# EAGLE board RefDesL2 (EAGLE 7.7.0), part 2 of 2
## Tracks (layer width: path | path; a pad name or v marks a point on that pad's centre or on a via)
AGND
  Top 0.152: 29.87,30.63 U2.A6 29.26,31.19 29.26,32 29.62,32.37 30.81,32.37 | C13.2 C15.2 C14.2 26.75,33.25 26.98,33.02 28.35,33.02 28.5,33.17 28.5,33.98 28.93,34.42 U2.A9 30.35,34.42 30.48,34.29 30.48,34.28 30.54,34.22 30.54,32.63 | 30.81,32.37 34.14,32.37 U2.E8 | 30.54,32.63 30.81,32.37 | 30.54,32.63 30.54,32.37
ANLG0  (via drill 0.3 pad 0.61)
  Top 0.152: v26.06,46.63 25.6,46.63 24.69,47.55 24.69,54.56 24.13,55.12 X6.1 | U2.B6 30.5,31.22 v30.5,31.47
  Bottom 0.152: v26.06,46.63 25.6,46.18 25.6,32.61 26.98,31.24 30.28,31.24 v30.5,31.47
CGND
  Top 0.381: X3.CGND1 X3.CGND2 X3.CGND3 X3.CGND4 | 17.42,15.27 X5.CGND5 | X5.CGND5 17.43,14.39 18.54,13.28 21.39,13.28 22.1,12.57 22.1,11.11 X5.CGND4 | 0.99,12.39 0.99,12.4 X5.CGND1 9.37,12.4 9.86,12.88 9.86,14.86 10.26,15.27 11.42,15.27 X5.CGND6 X5.CGND5
  Top 0.762: R2.1 4.7,63.88
  pour Top: 0,44.45 0,69.85 63.5,69.85 63.5,38.1 62.23,38.1 62.23,41.53 57.91,41.53 57.91,43.81 62.23,43.81 62.23,49.99 57.91,49.99 57.91,52.32 62.23,52.32 62.23,63.5 58.45,63.5 57.15,64.72 57.15,68.58 6.35,68.58 6.35,64.77 5.08,63.5 1.27,63.5 1.27,44.45
  pour Top: 0,44.45 1.27,44.45 1.27,6.35 5.08,6.35 6.35,5.08 6.35,2.03 23.44,2.03 23.44,1.27 41.53,1.27 41.53,11.66 42.27,12.4 44.42,12.4 45.77,11.13 54.56,11.13 55.75,12.4 57.71,12.4 58.47,11.43 62.23,11.43 62.23,38.1 63.5,38.1 63.5,0 0,0
  pour Bottom: 0,44.45 0,69.85 63.5,69.85 63.5,38.1 62.23,38.1 62.23,63.5 58.42,63.5 57.15,64.77 57.15,68.58 6.35,68.58 6.35,64.77 5.08,63.5 1.27,63.5 1.27,44.45
  pour Bottom: 0,44.45 1.27,44.45 1.27,6.35 5.08,6.35 6.35,5.08 6.35,1.27 41.53,1.27 41.53,11.66 42.29,12.4 44.42,12.4 45.75,11.15 45.77,11.13 54.56,11.13 54.56,11.1 55.75,12.4 57.68,12.4 58.45,11.43 62.23,11.43 62.23,38.1 63.5,38.1 63.5,0 0,0
ECAP_PWM0  (via drill 0.3 pad 0.61)
  Top 0.152: v29.34,37.52 29.01,37.85 25.2,37.85 24.84,37.49 24.84,32.97 24.13,32.26 X6.16 | U2.C18 31.8,45.26 v31.7,45.26
  Bottom 0.152: v31.7,45.26 31.7,40.39 33.68,38.41 33.68,37.03 32.31,35.66 30.63,35.66 29.34,36.96 v29.34,37.52
EMMC_RSTN  (via drill 0.3)
  Top 0.152: U2.R14 47.62,40.26 46.99,39.62 46.99,37.85 46.74,37.59 45.97,37.59 45.72,37.34 v45.72,32.64 | U9.K5 v27.97,9.34 | v27.96,9.35 v27.97,9.34 | R45.1 27.91,9.4 v27.97,9.34
  Bottom 0.152: v27.97,9.34 28.78,10.15 28.78,16.97 29.39,17.58 36.85,17.58 39.17,19.89 39.17,24.31 40.51,25.65 42.67,25.65 45.34,28.32 45.34,31.75 45.72,32.13 v45.72,32.64
GND  (via drill 0.3, 0.3 pad 0.61, 0.38, 0.38 pad 0.61, 0.76)
  Top 0.152: v44.04,57.76 43.89,57.76 43.23,58.42 C8.2 | v27.05,58.29 26.8,58.04 R26.1 | v29.26,45.41 29.26,45.72 29.39,45.85 U2.A18 | v26.92,25.02 27,25.09 R6.2 | U2.A1 29.26,24.84 v29.11,24.84 | U9.G5 30.71,10.84 | U9.N5 U9.P6 31.27,7.28 v31.27,6.55 | v30.48,6.55 30.48,7.07 U9.P4 | v23.24,16.64 C19.2 | U9.N2 28.33,7.84 27.94,8.23 v27.94,8.26 | U1.1 57.94,16.1 57.58,15.75 R1.1 v57.58,14.53 | v56.01,17.02 U1.TH | U9.C4 30.2,11.03 | R62.1 v57.25,50.42 | R61.1 v55.5,50.42 | v30.38,65.58 31.04,65.58 R39.1 | v45.59,45.21 45.72,45.21 U2.P17
  Top 0.254: U3.4 50.92,16.54 50.98,16.54 | C2.2 51,16.61 | v55.12,47.73 55.55,47.3 U5.4 | U9.H10 32.97,10.34 32.72,10.59 v31.95,10.59 | v31.95,10.59 31.14,10.59 30.89,10.84 U9.G5 30.38,10.84 30.2,11.02 30.2,11.03 | U9.K8 32.2,9.51 31.96,9.76 v31.96,10.59 v31.95,10.59 | U9.E7 31.7,11.76 31.95,11.51 v31.95,10.59 | 50.98,16.61 C2.2 | v51.92,16.54 50.98,16.54 | 50.98,16.54 C2.2 | R15.2 R57.2 | R57.2 R58.2 R59.1 R60.1 v53.59,50.42 | v48.26,50.42 R57.2
  Top 0.305: v13.46,67.44 12.21,67.44 RESET.4 | POWER.1 12.27,62.33 v13.56,62.33 | 16.92,60.72 BTN2.4 17,60.73 v15.85,60.73 | 16.93,65.8 BTN1.4 17,65.81 v15.85,65.81 | R7.1 v42.06,20.17 | R16.1 v44.04,20.17 | R23.1 v46.02,20.17 | R18.1 v48.01,20.17 | R10.1 v55.93,20.17 | U4.3 25.11,66.67 v24.26,66.67 | U6.1 24.38,60.33 v23.09,60.33 | X4.8 v36.58,64.77 | X4.4 v34.04,64.77 | X4.16 v41.66,64.77 | X4.20 v44.2,64.77 | C10.2 38.35,58.5 v38.35,59.44 | v51.97,20.17 R14.1 | C18.1 v20.95,19.81
  Top 0.381: U2.W3 U2.W2 v52.07,24.89 U2.V1 | RESET.2 RESET.4 | POWER.3 POWER.1 | BTN2.4 BTN2.2 | BTN1.4 BTN1.2 | X4.8 X4.10 X4.12 | R11.1 R14.1 R13.1 R12.1 | R7.1 R21.1 | R22.1 R23.1 R17.1 | R9.1 R10.1 | X3.GND | v30.35,2.92 C16.1 | v20.19,14.73 18.65,14.73 X5.GND | C9.1 v4.06,16.64 | C17.1 22.17,15.9 v21.46,15.9 | C11.2 v5.33,11.56 | C21.1 38.41,3.3 v37.72,3.3 | U7.2 v5.08,18.67 | v21.21,3.3 21.27,3.36 X5.6 | C20.1 40.72,6.27 v40.77,6.22 | C3.2 55.35,41.17 v55.12,41.4 | C12.2 v16,18.41
  Top 0.762: R2.2 v2.92,60.2
  other vias: 57.78,48.56 39.37,47.75 38.13,37.59 40.64,37.59 43.18,37.59 43.18,40.13 43.18,35 41.91,35.05 40.64,35.05 39.37,35.05 38.13,35.05 39.37,32.51 40.64,32.51 41.91,32.51 43.18,32.51 41.91,38.73 40.64,47.75 41.91,47.75 35.69,47.75 53.34,47.75 53.34,38.86 53.34,36.32 38.13,36.32 38.13,33.76 40.64,33.78 40.64,36.32 53.39,43.97 53.39,45.21 48.26,47.75 53.14,32.46 39.4,31.24 40.64,31.24 43.18,31.24 44.45,36.32 44.45,40.13 59.97,12.95 61.06,12.95 55.24,17.78 56.01,17.78 55.24,17.02 53.14,33.81 57.78,49.28
  pour Route15: -2.54,72.39 66.04,72.39 66.04,-2.54 -2.54,-2.54
  pour Top: 45.09,41.4 43.18,41.4 43.18,40.13 41.91,40.13 41.91,38.86 37.34,38.86 37.34,37.59 36.83,37.59 36.83,33.78 36.2,33.78 36.2,32.51 38.1,32.51 38.1,29.97 44.45,29.97 44.45,31.24 45.09,31.24 45.09,37.59 44.45,37.59 44.45,40.13 45.09,40.13
  pour Top (rank 2): 52.7,29.34 53.34,29.34 53.34,31.75 54.36,31.75 54.36,32 53.34,32 53.34,35.69 53.98,35.69 53.98,48.39 52.7,48.39 52.7,47.75 48.9,47.75 48.9,48.39 34.92,48.39 34.92,47.12 50.29,47.12 51.44,45.85 52.7,45.85
  pour Top (no thermals): 59.05,15.62 61.85,15.62 61.85,12.57 59.05,12.57
  pour Top (no thermals): 57.15,49.61 58.42,49.61 58.42,48.64 58.55,48.51 60.07,48.51 60.07,48.01 58.46,48.01 58.17,48.29 57.16,48.29
I2C0_SCL  (via drill 0.3 pad 0.61)
  Top 0.152: U2.C20 v31.7,49.07 32.18,49.55 R4.1 | v33.07,43.89 32.97,43.89 U2.C16 31.9,42.82 31.9,41.53 31.62,41.25 30.78,41.25 30.48,40.95 30.48,40.51 30.25,40.28 29.36,40.28 28.83,39.75 4.12,39.75 1.93,37.57 1.93,20.42 2.67,19.68 3.84,19.68 3.85,19.67 U7.1
  Bottom 0.152: v33.07,43.89 32.77,44.2 32.77,46.33 31.7,47.4 v31.7,49.07
I2C0_SDA
  Top 0.152: U2.C19 33.07,46.43 33.07,46.33 | 33.07,46.33 33.07,46.18 | 33.07,46.18 33.07,46.02 | 33.07,46.02 33.07,45.26 U2.C17 31.6,43.79 31.6,41.73 31.42,41.55 29.94,41.55 28.52,40.13 4.06,40.13 1.63,37.69 1.63,18.19 2.03,17.78 3.84,17.78 3.85,17.77 U7.3 | 33.38,46.33 33.53,46.48 33.83,46.48 34.29,46.94 34.29,47.55 34.14,47.7 33.5,47.7 33.17,48.03 33.17,49.91 33.35,50.09 R3.1 | 33.38,46.33 33.22,46.18 | 33.22,46.18 33.07,46.02 | 33.07,46.18 33.22,46.18 | 33.07,46.33 33.38,46.33
I2C1_SCL  (via drill 0.3)
  Top 0.152: v35.53,45.14 34.98,44.58 U2.E17 | X6.12 10.72,30.15 5.51,30.15 5.08,29.72 I2C1_SCL.TP
  Bottom 0.152: v35.53,45.14 35.53,45.62 36.17,46.25 36.17,47.02 36.35,47.19 36.35,48.18 35.41,49.12 35.41,55.55 35.74,55.88 37.36,55.88 38.02,56.54 44.65,56.54 45.31,57.2 45.31,62.33 45.03,62.61 45.03,65.28 43.84,66.47 30.02,66.47 21.61,58.06 11.05,58.06 8.99,56.01 8.99,31.52 9.6,30.91 11.48,30.91 X6.12
I2C1_SDA  (via drill 0.3)
  Top 0.152: U2.E18 v35.56,46.48 | X6.11 8.53,30.5 3.58,30.5 3.05,29.97 I2C0_SDA.TP
  Bottom 0.152: v35.56,46.48 35.1,46.94 35.1,55.7 35.61,56.21 37.19,56.21 37.82,56.84 44.48,56.84 44.98,57.35 44.98,62.13 44.73,62.38 44.73,65.13 43.69,66.17 30.2,66.17 21.74,57.71 12.42,57.71 11.66,56.95 11.66,33.63 X6.11
JTAG_EMU0  (via drill 0.3 pad 0.61)
  Top 0.152: 40.54,61.58 X4.13 40.39,59.56 40.56,59.38 R27.1 40.56,58.09 v40.23,57.76 | U2.C14 32.61,41 33.2,41 33.66,41.45 33.86,41.45 34.14,41.73 34.14,45.06 v34.27,45.19
  Bottom 0.152: v40.23,57.76 37.64,57.76 36.73,56.84 35.2,56.84 34.49,56.13 34.49,45.41 v34.27,45.19
JTAG_EMU1  (via drill 0.3 pad 0.61)
  Top 0.152: v33.05,41.6 32.77,41.6 32.61,41.45 32.31,41.45 31.62,40.77 U2.B14 | X4.14 v40.39,64.92 41.15,64.16 44.5,64.16 45.16,64.82 R42.1
  Bottom 0.152: v33.05,41.6 33.22,41.6 33.98,42.37 33.98,44.35 33.38,44.96 33.38,46.63 33.07,46.94 33.07,55.63 34.59,57.15 36.42,57.15 37.8,58.52 43.99,58.52 44.37,58.9 44.37,61.77 43.81,62.33 41,62.33 40.39,62.94 v40.39,64.92
JTAG_EMU2  (via drill 0.3 pad 0.61)
  Top 0.152: v23.32,41.91 23.32,41.76 23.98,41.1 25.73,41.1 R44.2 | v42.93,59.44 X4.17
  Bottom 0.152: v23.32,41.91 23.32,48.77 25.3,50.75 25.3,59.33 26.16,60.2 36.42,60.2 36.73,60.5 41.86,60.5 v42.93,59.44
JTAG_EMU3  (via drill 0.3 pad 0.61)
  Top 0.152: v42.93,64.9 X4.18 | U2.D14 33.93,41.05 v34.27,41.05
  Bottom 0.152: v34.27,41.05 34.27,41.66 34.44,41.83 34.44,44.12 34.8,44.48 34.8,55.88 35.46,56.54 37.03,56.54 37.64,57.15 44.35,57.15 44.68,57.48 44.68,62 42.93,63.75 v42.93,64.9
JTAG_TCK  (via drill 0.3 pad 0.61)
  Top 0.152: 29.87,38.25 U2.A12 29.18,38.23 v28.96,38.46 | v37.11,59.44 37.49,59.44 37.85,59.79 X4.9
  Top 0.381: X4.9 X4.11
  Bottom 0.152: v37.11,59.44 36.73,59.44 36.27,59.89 31.55,59.89 28.19,56.54 28.19,46.63 26.21,44.65 26.21,40.69 26.82,40.08 28.19,40.08 28.96,39.32 v28.96,38.46
JTAG_TDI  (via drill 0.3 pad 0.61)
  Top 0.152: v35.36,58.52 34.04,59.84 X4.3 | U2.B11 31.7,37.54 v31.7,37.64
  Bottom 0.152: v31.7,37.64 31.7,38.86 30.79,39.78 29.41,39.78 28.5,40.69 27.13,40.69 26.82,41 26.82,44.35 28.8,46.33 28.8,56.24 31.39,58.83 34.59,58.83 34.9,58.52 v35.36,58.52
JTAG_TDO  (via drill 0.3 pad 0.61)
  Top 0.152: v36.12,59.28 36.58,59.74 X4.7 | U2.A11 30.38,37.49 v30.48,37.49
  Bottom 0.152: v30.48,37.49 31.24,38.25 31.24,38.86 30.63,39.47 29.26,39.47 28.35,40.39 26.98,40.39 26.52,40.84 26.52,44.5 28.5,46.48 28.5,56.39 31.7,59.59 35.2,59.59 35.51,59.28 v36.12,59.28
JTAG_TMS  (via drill 0.3 pad 0.61)
  Top 0.152: U2.C11 v33.07,37.64 | v34.59,58.06 32.77,59.89 X4.1
  Bottom 0.152: v33.07,37.64 33.07,38.41 31.09,40.39 31.09,46.79 30.33,47.55 30.33,55.47 32.92,58.06 v34.59,58.06 34.14,58.06
JTAG_TRSTN  (via drill 0.3 pad 0.61)
  Top 0.152: v29.72,55.78 29.72,66.57 29.97,66.83 R39.2 X4.2 | U2.B10 31.7,36.27 v31.85,36.27
  Bottom 0.152: v31.85,36.27 31.85,36.88 32.31,37.34 32.31,38.71 30.94,40.08 29.57,40.08 28.65,41 27.43,41 27.13,41.3 27.13,44.2 29.11,46.18 29.11,55.17 v29.72,55.78
LCD_DATA0
  Top 0.152: R23.2 46.02,22.66 U2.R1
LCD_DATA1
  Top 0.152: R22.2 45.06,22.07 45.06,22.96 45.41,23.32 46.18,23.32 46.94,24.08 46.94,24.28 47.24,24.59 47.24,25.15 U2.R2
LCD_DATA2
  Top 0.152: R21.2 43.05,23.14 43.38,23.47 43.89,23.47 44.5,24.08 44.5,24.69 44.81,24.99 45.41,24.99 45.8,25.38 45.8,25.76 46.23,26.19 47.02,26.19 U2.R3
LCD_DATA3  (via drill 0.3 pad 0.61)
  Top 0.152: R20.1 v41.07,22.91 41.91,23.75 41.91,24.51 42.29,24.89 42.93,24.89 43.18,25.15 43.18,25.91 43.43,26.16 44.07,26.16 44.45,26.54 44.45,27.18 44.7,27.43 45.59,27.43 45.85,27.69 45.85,28.32 46.23,28.7 47.12,28.7 47.62,28.19 U2.R4
LCD_DATA4
  Top 0.152: R19.1 49,24.16 U2.T1
LCD_DATA5
  Top 0.152: R18.2 48.01,22.71 48.41,23.11 48.41,25.04 U2.T2
LCD_DATA6
  Top 0.152: R17.2 47.02,22.84 48.11,23.93 48.11,26.01 U2.T3
LCD_DATA7
  Top 0.152: R16.2 44.04,23.01 44.65,23.62 45.57,23.62 45.72,23.77 45.72,24.54 46.02,24.84 46.79,24.84 46.94,24.99 46.94,25.58 47.42,26.06 47.7,26.06 48.31,26.67 48.31,27.48 U2.T4
LCD_DATA8
  Top 0.152: 51.94,22.07 R14.2 51.97,22.66 51.84,22.78 51.13,22.78 50.16,23.75 U2.U1
LCD_DATA9
  Top 0.152: 50.98,22.4 R13.2 50.98,22.43 49.68,23.72 49.68,25.04 U2.U2
LCD_DATA10
  Top 0.152: R12.2 49.99,22.81 49.38,23.42 49.38,26.01 U2.U3
LCD_DATA11
  Top 0.152: R11.2 52.96,22.86 52.7,23.11 51.26,23.11 50.65,23.72 50.65,27.58 U2.U4
LCD_DATA12
  Top 0.152: R10.2 55.93,23.22 55.7,23.44 51.46,23.44 50.95,23.95 50.95,25.04 U2.V2
LCD_DATA13  (via drill 0.3 pad 0.61)
  Top 0.152: U2.V3 51.97,26.26 v51.97,26.21 | v54.94,22.91 R9.2
  Bottom 0.152: v54.94,22.91 54.94,25.38 54.1,26.21 v51.97,26.21
LCD_DATA14  (via drill 0.3 pad 0.61)
  Top 0.152: v53.95,22.91 R8.1 | U2.V4 51,28.5 v51,28.73
  Bottom 0.152: v53.95,22.91 53.95,25.3 53.65,25.6 51.51,25.6 51,26.11 v51,28.73
LCD_DATA15  (via drill 0.3 pad 0.61)
  Top 0.152: R7.2 v42.06,22.91 43.18,24.03 43.18,24.38 43.69,24.89 44.07,24.89 44.45,25.27 44.45,25.78 44.83,26.16 45.47,26.16 45.85,26.54 45.85,27.05 46.23,27.43 47.75,27.43 48.26,27.94 48.26,28.83 48.77,29.34 U2.T5
LDO_PGOOD  (via drill 0.3 pad 0.61)
  Top 0.152: U2.B5 31.14,29.36 v30.63,29.87 | 29.87,49.53 25.91,49.53 25.45,49.07 v25.45,48.92 | 29.87,49.53 30.02,49.38 | 29.87,49.53 30.02,49.68 | 30.02,49.68 30.33,49.99 30.33,50.93 30.86,51.46 LPGD.TP | 30.02,49.38 30.02,49.68 | U2.B20 31.01,48.39 30.02,49.38
  Bottom 0.152: v30.63,29.87 29.26,29.87 28.8,30.33 26.52,30.33 24.69,32.16 24.69,48.46 25.15,48.92 v25.45,48.92
MBUS_INT  (via drill 0.3, 0.38)
  Top 0.152: 48.87,35.71 U2.T10 48.39,35.69 47.9,36.17 47.17,36.17 v47.04,36.3 | v34.37,37.62 35.1,37.62 35.41,37.92 35.41,38.79 35.64,39.01 36.5,39.01 36.68,39.19 36.68,40.16 36.8,40.28 37.72,40.28 37.95,40.51 37.95,41.1 38.25,41.4 v39.45,41.4
  Bottom 0.152: X6.15 21.61,31.09 24.84,31.09 28.35,27.58 29.72,27.58 30.18,28.04 33.22,28.04 33.83,27.43 35.59,27.43 36.02,27.86 36.02,31.19 35.15,32.05 35.15,36.83 v34.37,37.62 | v39.45,41.4 39.45,40.26 40.18,39.52 42.32,39.52 45.54,36.3 v47.04,36.3
MBUS_RST  (via drill 0.3, 0.38)
  Top 0.152: U2.U10 49.63,36.22 48.62,36.22 v48.34,36.5 | v34.34,36.3 35.53,36.3 35.71,36.47 35.71,38.56 35.87,38.71 36.63,38.71 36.98,39.06 36.98,39.85 37.11,39.98 40.44,39.98 40.56,40.11 v40.69,40.11
  Bottom 0.152: X6.2 23.01,52.55 23.01,42.82 22.55,42.37 22.55,41.45 24.38,39.62 24.38,32 28.5,27.89 29.57,27.89 30.02,28.35 33.53,28.35 34.06,27.81 35.41,27.81 35.64,28.04 35.64,31.01 34.8,31.85 34.8,35.84 v34.34,36.3 | v40.69,40.11 42.22,40.11 45.49,36.83 47.62,36.83 47.95,36.5 v48.34,36.5
MMC0_CD  (via drill 0.3, 0.3 pad 0.61)
  Top 0.152: v33.02,42.67 U2.C15 | v43.84,59.41 44.2,59.77 X4.19 | 8.89,15.75 v8.89,16.13 X5.CD 7.13,14.75 5.97,13.59 R28.1
  Bottom 0.152: v43.84,59.41 43.84,59.16 43.51,58.83 37.64,58.83 36.27,57.45 34.44,57.45 32.77,55.78 32.77,46.79 33.07,46.48 33.07,44.65 33.68,44.04 33.68,43.33 v33.02,42.67 32,41.66 32,40.51 33.91,38.61 34.62,38.61 35.46,37.77 35.46,32.44 36.73,31.17 36.73,21.64 36.12,21.03 10.57,21.03 8.89,19.36 v8.89,16.13
MMC0_CLKO  (via drill 0.3, 0.3 pad 0.61)
  Top 0.152: U2.G17 37.54,44.58 v38.1,45.14 | X5.5 22.1,2.64 | R33.1 X5.5 | v19.3,2.67 X5.5
  Bottom 0.152: v38.1,45.14 38.1,44.7 37.16,43.76 37.16,42.29 38.25,41.2 38.25,39.73 36.98,38.46 36.98,33.17 38.25,31.9 38.25,20.9 36.22,18.87 20.09,18.87 18.75,17.53 18.75,3.12 19.2,2.67 v19.3,2.67
MMC0_CMD  (via drill 0.3, 0.3 pad 0.61)
  Top 0.152: U2.G18 v38.05,46.43 | X5.3 | 7.64,3.33 X5.3 | R32.1 8.26,9.14 10.16,7.24 10.16,3.56 v9.91,3.3 7.66,3.3 X5.3
  Bottom 0.152: v38.05,46.43 38.05,45.87 36.83,44.65 36.83,42.11 37.95,41 37.95,40.03 36.68,38.76 36.68,33.02 37.95,31.75 37.95,21.03 36.09,19.18 11.05,19.18 10.16,18.29 10.16,3.56 v9.91,3.3
MMC0_DAT0  (via drill 0.3, 0.3 pad 0.61)
  Top 0.152: U2.G16 v38.1,43.94 | v20.07,4.06 X5.7 22.61,4.06 22.86,3.81 R34.1
  Bottom 0.152: v38.1,43.94 38.1,43.43 37.47,42.8 37.47,42.44 38.56,41.35 38.56,39.55 37.29,38.28 37.29,33.35 38.56,32.08 38.56,20.75 36.35,18.54 20.24,18.54 19.13,17.42 19.13,4.37 19.43,4.06 v20.07,4.06
MMC0_DAT1  (via drill 0.3, 0.3 pad 0.61)
  Top 0.152: 22.1,4.75 X5.8 | U2.G15 37.54,42.04 v38.23,42.72 | R35.1 23.13,4.76 X5.8 | v20.57,4.7 22.05,4.7 X5.8
  Bottom 0.152: v20.57,4.7 20.04,4.7 19.51,5.23 19.51,17.32 20.37,18.19 36.45,18.19 38.86,20.6 38.86,32.23 37.59,33.5 37.59,38.15 38.86,39.42 38.86,42.09 v38.23,42.72
MMC0_DAT2  (via drill 0.3, 0.3 pad 0.61)
  Top 0.152: X5.1 7.62,4.78 v9.04,4.78 9.22,4.95 9.22,6.2 8.31,7.11 R31.1 | v36.78,46.41 36.22,45.85 U2.F18
  Bottom 0.152: v9.04,4.78 9.22,4.95 9.22,15.65 9.42,15.85 9.42,16.38 9.22,16.59 9.22,19.13 10.82,20.73 36.3,20.73 37.03,21.46 37.03,31.29 35.76,32.56 35.76,41.94 36.14,42.32 36.14,45.77 v36.78,46.41
MMC0_DAT3  (via drill 0.3, 0.3 pad 0.61)
  Top 0.152: U2.F17 36.7,45.09 v36.7,45.29 | X5.2 v9.52,4.06 | R36.1 8.05,8.13 9.73,6.45 9.73,4.27 v9.52,4.06 | v9.52,4.06 v9.53,4.06
  Bottom 0.152: v36.7,45.29 36.7,45.09 36.52,44.91 36.52,42.11 36.07,41.66 36.07,32.69 37.34,31.42 37.34,21.34 36.42,20.42 11.18,20.42 9.73,18.97 9.73,4.27 v9.52,4.06
MMC1_CLK
  Top 0.152: U9.M6 33.27,6.27 R46.1 R56.2
MMC1_CMD  (via drill 0.3, 0.3 pad 0.61)
  Top 0.152: U2.V9 51.44,34.34 51.38,34.34 v50.85,33.81 | U9.M5 31.71,7.33 33.33,5.71 38.73,5.71 38.99,5.97 38.99,14.22 v39.5,14.73 R47.1
  Bottom 0.152: v50.85,33.81 50.85,33.43 50.32,32.89 50.32,32.26 48.16,30.1 48.16,26.95 44.6,23.39 44.6,19.07 40.26,14.73 v39.5,14.73
MMC1_DAT0  (via drill 0.3, 0.3 pad 0.61)
  Top 0.152: 50.16,31.85 U2.U7 v49.61,32.44 | U9.A3 29.7,15.22 29.84,15.37 v32.64,15.37 33.78,15.37 34.16,15.75 34.16,16.51 32.94,17.73 R48.1
  Bottom 0.152: v32.64,15.37 40.26,15.37 43.23,18.34 43.23,22.5 47.83,27.1 47.83,30.3 49.61,32.08 v49.61,32.44
MMC1_DAT1  (via drill 0.3, 0.3 pad 0.61)
  Top 0.152: U2.V7 51.41,31.88 v50.88,31.34 | U9.A4 30.2,14.55 30.2,14.58 v30.45,14.83 | v41.02,14.73 40.77,14.73 40.51,14.48 R49.1
  Bottom 0.152: v50.88,31.34 50.34,31.34 48.79,29.79 48.79,26.59 45.21,23.01 45.21,17.65 42.29,14.73 v41.02,14.73 40.26,13.97 38.99,13.97 38.12,14.83 v30.45,14.83
MMC1_DAT2  (via drill 0.3, 0.3 pad 0.61)
  Top 0.152: 47.62,33.1 U2.R8 v46.89,33.88 | U9.A5 30.7,14.29 31.42,15.01 32.11,15.01 32.28,14.83 34.21,14.83 35.51,16.13 v35.51,16.99 34.77,17.73 R50.1
  Bottom 0.152: v46.89,33.88 46.89,32.13 46.13,31.37 46.13,27.94 43.08,24.89 40.89,24.89 39.78,23.77 39.78,18.82 37.95,16.99 v35.51,16.99
MMC1_DAT3  (via drill 0.3, 0.3 pad 0.61)
  Top 0.152: U2.T8 48.9,33.1 48.87,33.1 v48.31,33.66 | U9.B2 28.7,13.84 28.7,15.8 v29.36,16.46 29.36,17.91 29.77,18.31 37.8,18.31 38.33,17.78 42.42,17.78 42.8,17.4 R51.1
  Bottom 0.152: v48.31,33.66 48.21,33.66 47.78,33.22 47.78,31.9 46.76,30.89 46.76,27.58 43.31,24.13 41.27,24.13 40.39,23.24 40.39,17.68 39.17,16.46 v29.36,16.46
MMC1_DAT4  (via drill 0.3, 0.3 pad 0.61)
  Top 0.152: U2.U8 50.14,33.15 v49.66,33.63 | U9.B3 29.21,13.84 29.21,15.65 29.46,15.9 v33.33,15.9 32.21,17.02 30.61,17.02 30.35,17.27 R52.1
  Bottom 0.152: v49.66,33.63 49.66,33.48 48.49,32.31 48.49,31.57 47.47,30.56 47.47,27.28 42.93,22.73 42.93,18.59 40.23,15.9 v33.33,15.9
MMC1_DAT5  (via drill 0.3, 0.3 pad 0.61)
  Top 0.152: U2.V8 51.41,33.15 v50.88,32.61 | R53.1 41.58,13.89 41.66,13.97 41.66,15.24 v41.78,15.37 | v44.2,17.91 43.94,18.16 40.01,18.16 38.68,19.48 35.76,19.48 35.56,19.28 34.75,19.28 34.54,19.48 28.63,19.48 26.9,17.75 26.9,13.01 28.07,11.84 28.7,11.84 29.19,12.33 29.71,12.85 | 29.71,12.85 U9.B4 | 29.71,12.85 | 29.71,12.85
  Bottom 0.152: v50.88,32.61 50.88,32.33 48.49,29.95 48.49,26.77 44.91,23.19 44.91,18.41 44.4,17.91 v44.2,17.91 41.78,15.49 v41.78,15.37
MMC1_DAT6  (via drill 0.3, 0.3 pad 0.61)
  Top 0.152: 47.62,34.34 U2.R9 47.62,34.47 v47.02,35.08 | 30.71,13.37 30.71,13.34 U9.B5 31.2,13.84 31.2,14.21 31.52,14.53 34.62,14.53 v37.69,17.6 37.57,17.73 R54.1
  Bottom 0.152: v47.02,35.08 46.76,35.08 46.35,34.67 46.35,32.16 45.74,31.55 45.74,28.22 42.8,25.27 40.64,25.27 39.47,24.11 39.47,19.38 v37.69,17.6
MMC1_DAT7  (via drill 0.3, 0.3 pad 0.61)
  Top 0.152: U2.T9 v48.34,34.98 | U9.B6 | U9.B6 31.22,13.34 | U9.B6 31.7,13.84 31.7,13.87 32.05,14.22 36.07,14.22 v38.86,17.02 41.68,17.02 42.32,16.38 42.32,14.45 42.55,14.22 44.2,14.22 44.45,14.48 44.45,16.51 44.15,16.82 R55.1
  Bottom 0.152: v48.34,34.98 48.34,34.54 47.37,33.58 47.37,32.08 46.46,31.17 46.46,27.79 43.18,24.51 41.15,24.51 40.08,23.44 40.08,18.19 38.91,17.02 v38.86,17.02
N$1
  Top 0.152: VPLL.P$1 25.65,23.62 34.01,23.62 34.14,23.75 34.14,27.15 33.86,27.43 33.45,27.43 33.17,27.71 33.17,29.54 33.66,30.02 34.14,30.02 34.44,30.33 34.44,31.39 U2.E7
N$2
  Top 0.152: VIO.P$1 21.18,23.01 36.37,23.01 36.68,23.32 36.68,28.52 37.01,28.85 44.73,28.85 45.09,29.21 U2.N5
N$3  (via drill 0.3 pad 0.61)
  Top 0.152: v55.93,25.15 55.93,24.69 55.5,24.26 U2.Y1
  Bottom 0.152: v55.93,25.15 55.93,25.35 53.85,27.43 53.85,29.72 54.48,30.35 57.53,30.35 BAT_V.P$1
N$4
  Top 0.152: U2.W1 53.21,24.26 53.72,23.75 57.53,23.75 58.42,24.64 BAT_T.P$1
N$5
  Top 0.152: VMPU.P$1 23.42,23.32 34.16,23.32 34.44,23.6 34.44,27.05 34.82,27.43 35.15,27.43 35.41,27.69 35.41,34.9 U2.F10
N$6
  Top 0.152: PWR.2 47.03,65.34 46.74,65.05 46.74,62.36 46.05,61.67 46.05,53.39 46.35,53.09 R15.1
N$7  (via drill 0.3 pad 0.61)
  Top 0.152: v33.07,26.06 29.49,26.06 29.08,25.65 26.8,25.65 26.54,25.91 23.37,25.91 VCORE.P$1 | v35.51,26.06 35.71,26.26 35.71,30.12 U2.F6
  Bottom 0.152: v33.07,26.06 v35.51,26.06
N$8  (via drill 0.3 pad 0.61)
  Top 0.152: VDDR.P$1 20.88,28.5 28.19,28.5 28.5,28.8 v29.11,28.8 | U2.E5 34.29,28.7 v34.29,28.5
  Bottom 0.152: v29.11,28.8 33.98,28.8 v34.29,28.5
N$9
  Top 0.381: U8.1 59.69,34.72 R41.2 R40.1
N$10
  Top 0.381: R43.1 61.04,38.18 60.65,37.78 Q1.B 59.67,37.69 U8.2
N$11  (via drill 0.3, 0.3 pad 0.61)
  Top 0.152: v31.85,27.28 32.61,27.28 32.87,27.53 32.87,29.69 33.02,29.84 v33.02,31.24
  Top 0.305: U2.D7 v33.02,31.24
  Bottom 0.152: v31.85,27.28 31.85,26.36 31.24,25.76 15.6,25.76 VRTC.P$1
N$12  (via drill 0.3 pad 0.61)
  Top 0.152: 1V8.P$1 18.64,28.8 27.3,28.8 v28.07,29.57 | U2.D10 34.29,35.05 34.29,33.86 v34.27,33.83
  Bottom 0.152: v28.07,29.57 29.26,29.57 29.57,29.26 33.2,29.26 33.93,30 33.93,33.5 v34.27,33.83
N$13
  Top 0.152: 26.1,59.19 R24.2 26.09,60.33 U6.2
N$14  (via drill 0.3, 0.3 pad 0.61)
  Top 0.152: 50.16,34.39 U2.U9 50.14,34.42 v49.63,34.92 | v40.01,16.48 38.35,14.83 R56.1
  Bottom 0.152: v49.63,34.92 49.4,34.92 49,34.52 49,33.3 48.13,32.44 48.13,31.7 47.09,30.66 47.09,27.41 42.62,22.94 42.62,19.1 v40.01,16.48
N$15
  Top 0.381: X3.VBUS 58.49,45.54 57.53,44.58 R25.2
  pour Top (no thermals): 56.01,44.07 56.01,45.09 57.78,45.09 58.42,45.72 60.07,45.72 60.07,45.34 58.67,45.34 57.4,44.07
N$16
  Top 0.152: R44.1 28.88,41.07 U2.A15
N$17
  Top 0.152: R59.2 51.08,52.5 50.44,53.14 49.28,53.14 46.97,55.45 46.97,61.16 47.65,61.85 47.65,63.78 47.95,64.08 50.32,64.08 50.9,64.67 52.32,64.67 52.45,64.8 D0.2
N$18
  Top 0.152: D1.2 53.72,64.69 53.39,64.36 51.05,64.36 50.47,63.78 48.28,63.78 48.01,63.5 48.01,61.72 47.3,61.01 47.3,55.63 49.45,53.47 50.55,53.47 50.95,53.06 52.35,53.06 52.91,52.5 R60.2
N$19
  Top 0.152: R61.2 55.5,53.24 55.24,53.49 52.12,53.49 50.67,54.94 48.87,54.94 48.08,55.73 48.08,60.12 49.07,61.11 55.32,61.11 55.96,61.75 55.96,63.55 54.99,64.52 D2.2
N$21  (via drill 0.3, 0.3 pad 0.61)
  Top 0.152: v22.25,67.67 22.06,67.47 BTN1.1 | U2.V17 50.85,45.16 50.85,45.87 50.09,46.63 41.05,46.63 40.64,46.23 40.64,43.18 41.15,42.67 v41.91,42.67
  Top 0.381: BTN1.3 BTN1.1
  Bottom 0.152: v22.25,67.67 22.55,67.97 46.02,67.97 47.35,66.65 47.35,50.77 42.55,45.97 42.55,44.2 42.55,44.17 42.55,43.31 v41.91,42.67
N$22
  Top 0.152: R62.2 57.25,53.24 56.69,53.8 52.27,53.8 50.83,55.24 49.02,55.24 48.39,55.88 48.39,59.94 49.25,60.81 55.47,60.81 56.26,61.59 D3.2
N$24
  Top 0.152: U2.B4 30.33,27.28 28.19,27.28 27.69,26.77 R6.1
N$34
  Top 0.152: 50.67,65.05 D5.2 50.67,64.87 50.22,64.41 47.8,64.41 47.35,63.96 47.35,62.03 46.66,61.34 46.66,55.24 49.4,52.5 R58.1
N$35
  Top 0.152: R57.1 48.26,52.98 46.35,54.89 46.35,61.52 47.04,62.2 47.04,64.47 47.3,64.72 49.25,64.72 49.39,64.86 49.39,65.35 D4.2
N$36  (via drill 0.3, 0.3 pad 0.61)
  Top 0.152: U2.U13 49.68,39.98 49.68,41.05 49.89,41.25 50.42,41.25 50.93,40.74 50.93,40.49 51.13,40.28 51.64,40.28 v52.05,39.88 | v60.73,57.89 v59.21,57.89 | D5.1 v50.67,67.84
  Bottom 0.152: v52.05,39.88 51.41,39.24 50.55,39.24 50.24,39.55 50.24,40.36 50.77,40.89 52.73,40.89 54.13,42.29 58.29,42.29 60.86,44.86 60.86,52.93 59.72,54.08 59.72,57.38 v59.21,57.89 | v50.67,67.84 51.56,67.84 57.45,61.95 59.33,61.95 60.35,60.94 60.35,58.27 v60.73,57.89
N$37  (via drill 0.3, 0.3 pad 0.61)
  Top 0.152: 50.11,40.72 U2.U14 50.8,40.13 v50.8,39.83 | D4.1 v49.4,67.84
  Bottom 0.152: v50.8,39.83 51.54,40.56 52.83,40.56 54.25,41.99 58.47,41.99 61.16,44.68 61.16,53.09 60.02,54.23 60.02,60.81 59.18,61.65 57.3,61.65 51.64,67.31 49.94,67.31 v49.4,67.84
N$38  (via drill 0.3, 0.3 pad 0.61)
  Top 0.152: BTN2.1 21.11,62.38 v22.1,62.38 | U2.U16 50.14,43.31 49.35,44.09 42.27,44.09 41.91,44.45 v41.91,45.21
  Top 0.381: BTN2.3 BTN2.1
  Bottom 0.152: v22.1,62.38 22.1,66.6 23.16,67.67 45.57,67.67 47.02,66.22 46.99,66.19 46.99,50.93 41.91,45.85 v41.91,45.21
N$52
  Top 0.152: WP.P$1 6.1,19.78 6.02,19.7 6.05,19.67 U7.5 | 7.66,19.27 R37.2
  Top 0.381: 7.66,19.27 7.12,19.27 6.71,19.67 6.66,19.62 U7.5
N$81  (via drill 0.3)
  Top 0.152: U9.C2 28.71,13.34 28.7,13.34 28.07,13.97 v28.07,15.52 | v26.29,16.64 C19.1
  Bottom 0.152: v28.07,15.52 28.07,16.15 27.58,16.64 v26.29,16.64
NINT  (via drill 0.3 pad 0.61)
  Top 0.152: NINT.TP v31.93,56.08 | U2.B19 31.75,46.48 | U2.B18 31.75,46.48 | 31.75,46.48 v31.85,46.48
  Bottom 0.152: 31.7,56.08 v31.93,56.08 31.55,56.08 30.63,55.17 30.63,47.7 v31.85,46.48
NWAKEUP  (via drill 0.3 pad 0.61)
  Top 0.152: U2.A19 28.8,48.16 v25.45,48.16 | 27.43,51.66 v27.28,51.66 27.53,51.66 NWKP.TP | v31.9,29.87 31.9,29.82 U2.C5
  Bottom 0.152: v27.28,51.66 27.28,49.07 26.36,48.16 v25.45,48.16 24.99,47.7 24.99,32.31 26.67,30.63 31.14,30.63 v31.9,29.87
OSC0_GND
  Top 0.305: U2.L20 42.55,49.53 | 42.55,49.53 41.96,50.11 C5.2 | 42.55,49.53 43.13,50.11 C4.2
OSC0_IN
  Top 0.152: U2.M20 43.81,49.53 44.25,49.96 C4.1 44.25,51.26 43.81,51.69 R29.2 43.1,53.65 43.31,53.85 Y1.P$2
OSC0_OUT
  Top 0.152: U2.K20 41.27,49.53 40.84,49.96 C5.1 40.84,51.28 41.25,51.69 R29.1 41.99,53.65 41.78,53.85 Y1.P$1
OSC1_GND
  Top 0.305: U2.G20 37.47,49.4 | 37.47,49.4 36.88,49.99 C7.2 | 37.47,49.4 38.05,49.99 C6.2
OSC1_IN
  Top 0.152: U2.H20 38.73,49.53 39.17,49.96 C6.1 39.17,51.38 38.73,51.82 R30.2 37.85,51.99 37.85,53.59 38.1,53.85 Y2.P$2
OSC1_OUT
  Top 0.152: U2.F20 36.2,49.53 35.76,49.96 C7.1 35.76,51.38 36.2,51.82 R30.1 37.08,51.99 37.08,53.59 36.83,53.85 Y2.P$1
PMIC_PGOOD  (via drill 0.3 pad 0.61)
  Top 0.152: v23.93,43.18 23.93,42.22 24.38,41.76 28.8,41.76 29.57,42.52 30.63,42.52 U2.B15 | U2.A20 29.46,48.77 v26.21,48.77 | U4.2 25.78,65.91 26.16,65.53 27.74,65.53 28.32,64.95 v28.32,59.44 PGD.TP
  Bottom 0.152: 24.69,49.68 23.62,48.62 23.62,43.48 v23.93,43.18 | 24.69,49.68 25.6,50.6 25.6,59.13 25.91,59.44 v28.32,59.44 | 24.69,49.68 25.76,49.68 26.21,49.23 v26.21,48.77
PWR_BUT
  Top 0.152: POWER.2 12.81,60.8 15.7,57.91 22.71,57.91 25.76,54.86 33.98,54.86 35.05,53.8 35.05,49.78 U2.D20
  Top 0.381: POWER.4 POWER.2
PWREN  (via drill 0.3 pad 0.61)
  Top 0.152: U2.C6 32.36,30.58 32.36,30.89 v31.85,31.39 | v25.91,47.55 28.19,47.55 29.41,46.33 30.18,46.33 30.48,46.63 30.48,47.24 30.94,47.7 32.69,47.7 | 32.87,47.88 33.05,47.7 | 32.69,47.7 32.87,47.88 | 32.87,47.88 32.87,48.77 32.77,48.87 32.77,51.82 PWREN.TP | 32.69,47.7 33.05,47.7 | U2.D19 33.63,47.12 33.05,47.7
  Bottom 0.152: v25.91,47.55 25.3,46.94 25.3,32.46 26.82,30.94 31.39,30.94 v31.85,31.39
RESET
  Top 0.152: RESET.3 13.68,65.88 14.94,64.62 23.18,64.62 25.46,62.34 U6.3 26.1,62.91 25.13,63.87 U4.4
  Top 0.381: RESET.1 RESET.3
SPI0_CS0
  Top 0.152: X6.3 18.9,55.12 20.52,53.49 22.1,53.49 24.08,51.51 24.08,47.24 26.36,44.96 27.89,44.96 29.54,43.31 U2.A16
SPI0_D0  (via drill 0.3 pad 0.61)
  Top 0.152: v27.89,43.28 27.13,43.28 27.12,43.28 27.03,43.28 23.32,46.99 23.32,50.9 21.79,52.43 16.54,52.43 13.84,55.12 X6.5 | U2.B17 v30.53,43.99
  Bottom 0.152: 28.35,43.28 v27.89,43.28 29.82,43.28 v30.53,43.99
SPI0_D1
  Top 0.152: X6.6 11.33,55.12 14.63,51.82 21.64,51.82 22.86,50.6 22.86,46.63 26.98,42.52 28.96,42.52 29.26,42.82 30.63,42.82 U2.B16
SPI0_SCLK  (via drill 0.3 pad 0.61)
  Top 0.152: 27.43,44.2 v27.89,44.2 26.67,44.2 23.62,47.24 23.62,51.21 21.95,52.88 18.57,52.88 16.33,55.12 X6.4 | v28.96,44.65 29.03,44.58 U2.A17
  Bottom 0.152: v27.89,44.2 28.35,44.65 v28.96,44.65
SYS_RESETN  (via drill 0.3 pad 0.61)
  Top 0.152: v28.65,37.03 28.65,36.88 U2.A10 | R24.1 R26.2 24.97,57.45 25.3,57.12 26.44,57.12 v26.67,56.9 26.67,55.78 27.28,55.17 32.61,55.17 33.4,55.96 WRST.TP 41.15,57.15 41.73,57.73 C8.1 41.66,58.5 X4.15
  Bottom 0.152: v28.65,37.03 28.19,37.49 28.19,39.62 28.04,39.78 26.67,39.78 25.91,40.54 25.91,44.81 27.89,46.79 27.89,56.41 27.41,56.9 v26.67,56.9
SYS_RTC_1P8V  (via drill 0.3, 0.3 pad 0.61, 0.38 pad 0.3)
  Top 0.305: v27.28,64.62 U4.5
  Top 0.381: v45.72,40.13 U2.P14 | R41.1 57.58,33.6 56.64,34.54 56.64,35.31 | v48.26,37.59 v50.8,37.59 | v57.02,37.08 57.53,37.08
  Bottom 0.381: v27.28,64.62 29.87,67.21 45.41,67.21 46.56,66.06 46.56,51.26 41.02,45.72 41.02,42.29 42.04,41.27 44.7,41.27 45.72,40.26 v45.72,40.13 45.72,38.86 46.99,37.59 v48.26,37.59 | 56.52,37.59 v57.02,37.08 56.26,37.85 51.05,37.85 v50.8,37.59
  pour Top: 57.78,34.8 57.78,39.88 56.39,39.88 56.39,34.8
SYS_VDD1_3P3V  (via drill 0.3, 0.3 pad 0.61, 0.38, 0.38 pad 0.61, 0.76)
  Top 0.152: R42.2 v45.72,63.02 | R27.2 39.52,58.5 v39.52,59.41 | v31.34,49.84 31.06,50.11 R4.2 | R3.2 34.44,50.7 34.44,51.16 34.29,51.31 v33.91,51.31 | U9.N4 U9.P3 v29.69,6.55 | U9.M4 U9.N4 | U9.J10 33.63,9.42 v33.63,8.94 33.1,8.94 32.72,9.32 32.72,9.33 U9.K9 | U9.J10 33.2,9.86 | U9.F5 31.23,11.34 v31.32,11.25 31.2,11.37 U9.E6 U9.C6 | U9.N4 U9.P5 | R5.2 v53.54,14.53 | 3.99,13.56 R28.2 v3.17,13.59 | 7.66,18.15 7.64,18.16 7.62,18.16 R37.1 | R45.2 v23.24,9.4 | v38.35,4.32 R46.2 | U9.J10
  Top 0.305: R20.2 v41.07,20.17 | R19.2 v49,20.17 | R8.2 v53.95,20.17 | X4.5 v35.31,63.5 | C10.1 v36.2,58.42 | U6.4 24.18,62.36 v23.24,62.36 | v17.78,19.81 C18.2
  Top 0.381: v34.49,2.92 C16.2 | v8.64,2.67 X5.4 | C17.2 22.15,17.14 v21.46,17.14 | R35.2 R34.2 R33.2 24.31,2.08 v24.26,2.03 | R31.2 R36.2 R32.2 v3.05,9.14 | C11.1 v3.56,11.56 | C21.2 38.41,2.03 v37.72,2.03 | R37.1 v7.62,17.27 | v6.99,16.64 C9.2 6.02,17.69 U7.4 | C20.2 40.69,5.16 v40.77,5.08 | R47.2 R49.2 R53.2 41.99,12.78 v42.42,13.21 | R51.2 42.8,15.37 v43.31,14.86 43.81,15.37 R55.2 | R54.2 R50.2 R48.2 R52.2 29.46,18.85 28.45,17.83 v28.45,17.53 | C12.1 v12.95,18.41
  other vias: 50.8,49.66
  pour Route2: -1.27,71.12 64.77,71.12 64.77,-1.27 -1.27,-1.27
  pour Top: 49.53,50.55 52.07,50.55 52.07,48.39 49.53,48.39
SYS_VDD2_3P3V  (via drill 0.3 pad 0.61)
  Top 0.152: 3V3_2.P$1 11.94,23.57 12.9,22.61 36.68,22.61 36.98,22.91 36.98,28.4 37.13,28.55 45.19,28.55 45.85,29.21 45.85,29.62 46.23,30 51.71,30 52.05,30.33 v52.05,36.27 | U2.Y11 v54.86,36.96 54.86,37.54 54.48,37.92 54.48,51.46 53.98,51.97 45.9,51.97 45.74,52.12 45.74,61.82 46.43,62.51 46.43,66.47 46.94,66.98 47.74,66.98 PWR.1
  Bottom 0.152: v52.05,36.27 52.73,36.96 v54.86,36.96
SYS_VOUT  (via drill 0.76)
  Top 0.305: SYS5V.P$1 10.67,25.91 10.67,24.08 13.89,20.85 38.43,20.85 40.34,18.95 58.64,18.95 59.17,19.48 v60.45,19.48
  Top 0.762: C1.+ v60.45,19.48
  Bottom 0.305: SYS5V.P$1 7.75,31.37 X6.10
  Bottom 0.762: v54.81,27.74 60.45,22.1 v60.45,19.48
  pour Top: 52.07,28.7 53.34,28.7 53.34,28.07 55.24,28.07 55.24,27.43 52.07,27.43
  pour Top (no thermals): 57.15,17.93 59.05,17.93 59.05,18.54 61.85,18.54 61.85,16.26 59.05,16.26 59.05,16.87 57.15,16.87
UART0_RX
  Top 0.152: U2.E15 34.44,42.52 34.44,43.64 34.7,43.89 35.36,43.89 35.71,43.54 35.71,39.52 35.18,38.99 18.52,38.99 17.91,38.38 X6.14
UART0_TX
  Top 0.152: U2.E16 34.92,42.9 35.41,42.42 35.41,40.32 35.06,39.98 29.62,39.98 29.01,39.37 16.26,39.37 15.37,38.48 X6.13
USB0_DM  (via drill 0.3 pad 0.61)
  Top 0.152: U2.N18 45.44,45.85 v45.7,46.1 | X3.D- 59.37,46.18 58.55,46.18 58.5,46.13 v57.78,46.13 57.63,46.13 57.48,46.28 56.99,46.28 | 56.88,46.28 56.99,46.28 | 56.99,46.28 U5.1
  Bottom 0.152: v57.78,46.13 57.66,46.13 57.43,46.35 56.01,46.35 55.75,46.1 55.75,45.72 55.63,45.59 55.24,45.59 55.12,45.72 55.12,46.1 54.86,46.35 54.61,46.35 54.36,46.1 54.36,45.72 54.23,45.59 53.85,45.59 53.72,45.72 53.72,46.1 53.47,46.35 53.21,46.35 52.96,46.1 52.96,45.72 52.83,45.59 52.45,45.59 52.32,45.72 52.32,46.1 52.12,46.3 45.9,46.3 v45.7,46.1
USB0_DP  (via drill 0.3 pad 0.61)
  Top 0.152: U2.N17 45.09,44.65 v44.6,45.14 | X3.D+ 59.35,46.81 58.55,46.81 58.47,46.89 v57.78,46.89 57.58,46.89 57.48,46.79 U5.2
  Bottom 0.152: v44.6,45.14 44.45,45.29 44.45,45.97 45.14,46.66 57.38,46.66 57.61,46.89 v57.78,46.89
USB0_ID  (via drill 0.3 pad 0.61)
  Top 0.152: X3.ID 58.46,47.49 58.19,47.75 57.81,47.75 v57.78,47.73 57.34,47.29 U5.3 | U2.P16 v45.72,42.67
  Bottom 0.152: v57.78,47.73 57.05,46.99 44.96,46.99 44.07,46.1 44.07,44.32 v45.72,42.67
USB1_DM  (via drill 0.3 pad 0.61)
  Top 0.152: U2.R18 47.62,45.77 v46.99,45.14
  Top 0.254: U3.1 49.92,13.74 X2.2
  Bottom 0.152: X2.2 49.16,13.48 50.01,14.33 50.01,27.05 49.73,27.33 49.73,29.08 50.55,29.9 52.68,29.9 54.3,31.52 54.3,34.7 53.87,35.13 50.85,35.13 49.28,36.7 49.28,43.51 48.21,44.58 47.55,44.58 v46.99,45.14
USB1_DP  (via drill 0.3 pad 0.61)
  Top 0.152: v48.08,45.14 47.62,44.68 U2.R17
  Top 0.254: U3.2 50.42,13.74 X2.3
  Bottom 0.152: X2.3 51.16,13.48 50.32,14.33 50.32,14.99 50.42,15.09 50.62,15.09 50.77,15.24 50.77,15.44 50.62,15.6 50.44,15.6 50.32,15.72 50.32,27.3 50.04,27.58 50.04,28.96 50.67,29.59 52.83,29.59 54.61,31.37 54.61,34.85 54.03,35.43 51.05,35.43 49.61,36.88 49.61,43.61 v48.08,45.14
USB1_DRVVBUS  (via drill 0.3, 0.3 pad 0.61)
  Top 0.152: U2.F15 36.78,41.45 v36.78,41.33 | U1.4 57.11,18.37 56.9,18.16 56.9,16.2 56.46,15.77 R1.2 56.46,13.74 54.28,11.56 46.15,11.56 44.96,12.75 44.96,18.03 44.45,18.54 40.13,18.54 38.79,19.89 v35.31,19.89
  Bottom 0.152: v36.78,41.33 36.78,39.34 36.37,38.94 36.37,32.87 37.64,31.6 37.64,21.18 36.35,19.89 v35.31,19.89
USB1_OCN  (via drill 0.3, 0.3 pad 0.61)
  Top 0.152: v55.55,15.37 R5.1 54.66,15.93 54.36,16.23 54.36,18.16 54.14,18.37 U1.5 53.27,18.34 v51.87,18.34 | v48.23,42.82 48.41,42.82 U2.T16
  Bottom 0.152: v51.87,18.34 50.62,19.58 50.62,27.51 50.34,27.79 50.34,28.83 50.8,29.29 52.96,29.29 54.91,31.24 54.91,35 54.18,35.74 51.21,35.74 49.94,37.01 49.94,44.81 50.19,45.06 50.19,45.54 49.76,45.97 46.53,45.97 46.13,45.57 46.13,44.63 46.81,43.94 47.88,43.94 48.54,43.28 48.54,42.95 48.41,42.82 v48.23,42.82
USB1_PWR
  Top 0.254: U3.6 49.92,16.59 C2.1 49.86,17.2 49.78,17.27
  pour Top (no thermals): 48.01,15.75 48.01,18.54 49.28,18.54 49.28,17.83 54.1,17.83 54.1,16.26 52.58,16.26 52.58,17.07 49.28,17.07 49.28,15.75
USB1_VBUS  (via drill 0.3, 0.3 pad 0.61)
  Top 0.152: U2.T18 48.95,45.85 v49.53,45.26 | v45.85,18.16 46.1,17.91 FB1.1
  Bottom 0.152: v49.53,45.26 49.12,45.67 46.71,45.67 46.46,45.41 46.46,44.81 46.99,44.27 48.01,44.27 48.95,43.33 48.95,36.55 50.67,34.82 53.65,34.82 54,34.47 54,31.7 52.53,30.23 50.37,30.23 49.4,29.26 49.4,27.18 49.68,26.9 49.68,20.09 48.9,19.3 46.99,19.3 v45.85,18.16
USB_DC  (via drill 0.3)
  Top 0.152: v15.62,21.67 38.28,21.67 40.62,19.33 58.19,19.33 59.94,21.08 59.94,25.78 60.33,26.16 61.21,26.16 62.36,27.3 62.36,32.38 61.82,32.92 54.63,32.92 | U2.P15 v45.72,41.4
  Top 0.254: U5.6 55.43,46.29 55.12,45.97 v55.12,44.32 55.12,43.56 55.88,42.8 R25.1
  Top 0.381: 56.77,43.18 56.77,42.42 56.64,42.29 | 54.86,34.42 55.24,34.42 55.75,34.92 55.75,40.26 56.01,40.51 56.9,40.51 57.07,40.69 C3.1 57.07,41.48 56.64,41.91 56.64,42.29 | 56.64,42.29 R25.1
  Bottom 0.152: USB5V.P$1 9.4,23.52 10.52,22.4 10.52,22.38 11.56,21.34 15.29,21.34 v15.62,21.67 | v45.72,41.4 43.31,43.81 43.31,46.1 44.7,47.5 46.35,47.5 47.37,48.51 52.07,48.51 53.38,49.82 58.68,49.82 59.18,49.32 59.18,45.59 57.91,44.32 v55.12,44.32
  pour Top: 53.98,35.05 54.86,35.05 54.86,32.51 53.98,32.51
USR0  (via drill 0.3)
  Top 0.152: U2.V15 51.44,42.06 v51.99,42.62 | D0.1 v52.45,67.87 | v59.13,57.02 v60.71,57.02
  Bottom 0.152: v52.45,67.87 52.45,67.44 57.63,62.26 59.51,62.26 60.68,61.09 60.68,58.73 61.29,58.12 61.29,57.4 60.91,57.02 v60.71,57.02 | v59.13,57.02 58.55,56.44 58.55,54.3 60.25,52.6 60.25,45.16 57.99,42.9 52.27,42.9 v51.99,42.62
USR1  (via drill 0.3)
  Top 0.152: U2.U15 v50.75,42.62 | D1.1 v53.72,67.87 | v59.18,58.8 v61.37,58.8
  Bottom 0.152: v50.75,42.62 51.33,43.2 57.81,43.2 59.94,45.34 59.94,52.27 58.24,53.98 58.24,57.86 v59.18,58.8 | v53.72,67.87 53.72,66.65 57.81,62.56 59.66,62.56 61.04,61.19 61.04,59.13 v61.37,58.8
USR2  (via drill 0.3)
  Top 0.152: 48.9,42.01 U2.T15 49,42.04 49.48,41.55 50.9,41.55 v51,41.45 | D2.1 v54.99,67.87 | v59.11,56.24 v60.73,56.24
  Bottom 0.152: v51,41.45 52.83,41.45 53.98,42.6 58.14,42.6 60.55,45.01 60.55,52.78 59.41,53.92 59.41,55.93 v59.11,56.24 | v54.99,67.87 54.99,65.86 57.99,62.87 59.87,62.87 61.34,61.39 61.34,59.69 61.9,59.13 61.9,57.4 v60.73,56.24
USR3  (via drill 0.3)
  Top 0.152: U2.V16 51.44,43.33 v51.99,43.89 | D3.1 v56.26,67.87 | v59.18,59.94 61.19,61.95 v61.19,62.46
  Bottom 0.152: v51.99,43.89 52.63,44.53 54.03,44.53 54.99,43.56 57.68,43.56 59.61,45.49 59.61,52.12 57.91,53.82 57.91,58.67 v59.18,59.94 | v56.26,67.87 56.26,65.05 58.14,63.17 60.48,63.17 v61.19,62.46
VBUS
  pour Top (no thermals): 46.23,17.02 47.5,17.02 47.5,12.06 46.1,12.06 45.85,12.32 45.85,14.1 46.23,14.61
VDD_3V3A  (via drill 0.38 pad 0.61)
  Top 0.381: v57.91,40.64 59.05,40.64 | v52.07,38.86 48.51,38.86 48.51,38.89 48.23,39.17 48.23,41.1 47.62,41.71 U2.R15 | R43.2 62.08,39.29 62.23,39.14 62.23,37.26 61.98,37.01 R40.2
  Bottom 0.381: v52.07,38.86 53.85,40.64 v57.91,40.64
  pour Top: 58.55,38.73 58.55,41.02 61.59,41.02 61.59,38.73
VDD_5V  (via drill 0.3, 0.76, 0.76 pad 0.61)
  Top 0.152: v14.48,21.97 14.99,21.97 15.24,22.23 38.23,22.23 40.82,19.63 57.99,19.63 59.56,21.21 59.56,26.04 60.07,26.54 61.09,26.54 62,27.46 62,32.23 61.72,32.51 57.76,32.51 56.79,31.55 v56.79,31.27
  Top 0.762: v61.16,54.79 54.74,54.79 51.49,58.04 X1.IN | v56.79,31.27 56.79,30.76 55.96,29.92 54.79,29.92
  Bottom 0.152: VDD5V.P$1 9.4,26.19 10.67,24.92 10.67,23.32 11.71,22.28 14.17,22.28 v14.48,21.97
  Bottom 0.762: v61.16,54.79 61.77,54.18 61.77,37.26 56.79,32.28 v56.79,31.27
  pour Top: 53.98,31.24 53.98,28.7 55.12,28.7 55.12,31.24
VDD_ADC
  Top 0.152: U2.D8 33.12,33.68 32,33.68 31.7,33.98 31.7,34.9 31.39,35.2 29.26,35.2 28.27,36.2 28.04,36.2 27.86,36.37 R38.2 27.86,37.06 27.58,37.34 26.36,37.34 26.06,37.03 26.06,32.16 26.52,31.7 28.04,31.7 29.84,29.9 U2.A5 U2.A4 29.52,27.74 28.04,27.74 27.48,27.18 VADC.P$1
VIN_BAT
  Top 0.381: 54.56,26.06 55.47,26.06 55.93,26.52 55.93,28.04 57.76,29.87 59.59,29.87 BAT5V.P$1
  pour Top: 53.34,24.89 53.34,26.8 55.24,26.8 55.24,24.89
VREFP_ADC
  Top 0.152: U2.B9 30.63,34.9 28.91,34.9 28.68,34.67 C15.1 | C14.1 C15.1 | C15.1 C13.1 27.43,35.69 27.3,35.81 27.3,36.55 27.15,36.7 R38.1

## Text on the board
tPlace: VS | 5V | SDA | SCL | BAT | TS | GND | I2C1
tNames: IO | USR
